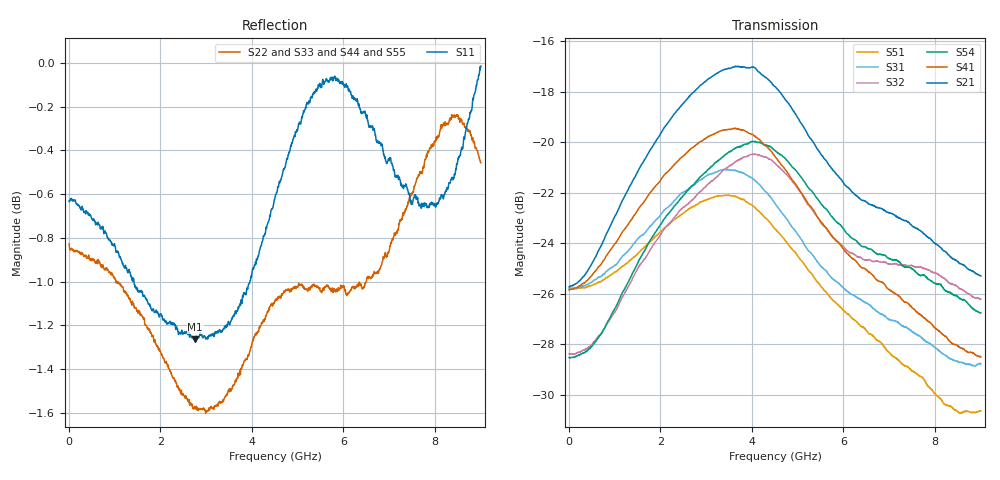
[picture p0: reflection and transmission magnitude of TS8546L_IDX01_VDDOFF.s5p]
# GHz S DB R 50
! CMT, SN0916, 25263762, 26.7.0
! Date: 16.07.2026 12:20:04
! Data: Format
! Freq S1.1:dB/Ang S1.2:dB/Ang S1.3:dB/Ang S1.4:dB/Ang S1.5:dB/Ang
!  S2.1:dB/Ang S2.2:dB/Ang S2.3:dB/Ang S2.4:dB/Ang S2.5:dB/Ang
!  S3.1:dB/Ang S3.2:dB/Ang S3.3:dB/Ang S3.4:dB/Ang S3.5:dB/Ang
!  S4.1:dB/Ang S4.2:dB/Ang S4.3:dB/Ang S4.4:dB/Ang S4.5:dB/Ang
!  S5.1:dB/Ang S5.2:dB/Ang S5.3:dB/Ang S5.4:dB/Ang S5.5:dB/Ang
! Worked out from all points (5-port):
!   2001 points, 10 MHz to 9 GHz, reference 50 ohm
!   strongest paths, dB at 10 MHz, 2.257 GHz, 4.505 GHz, 6.753 GHz, 9 GHz:
!     S21: -25.7, -19.0, -17.8, -22.6, -25.3
!     S41: -25.9, -21.0, -20.6, -25.5, -28.5
!     S54: -28.5, -22.7, -20.3, -24.4, -26.8
!     S32: -28.4, -23.1, -20.8, -24.7, -26.2
!     S31: -25.8, -22.4, -22.4, -26.7, -28.8
!     S51: -25.8, -23.1, -23.4, -27.9, -30.6
!   lowest |S11| = -1.3 dB at 2.761 GHz (marker M1), VSWR 13.77, Z = 5.6 + j36.7 ohm
!   |S11| at or under -10 dB: nowhere
